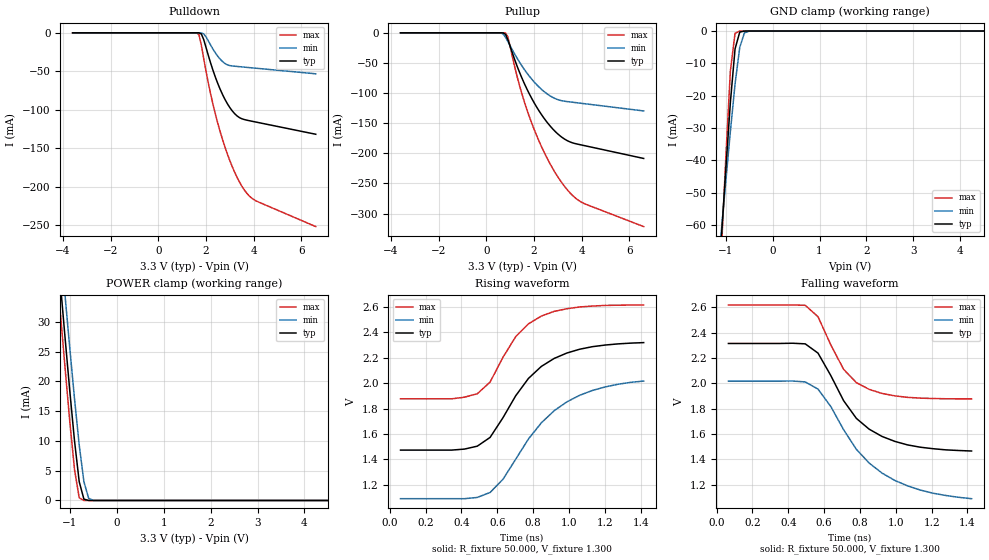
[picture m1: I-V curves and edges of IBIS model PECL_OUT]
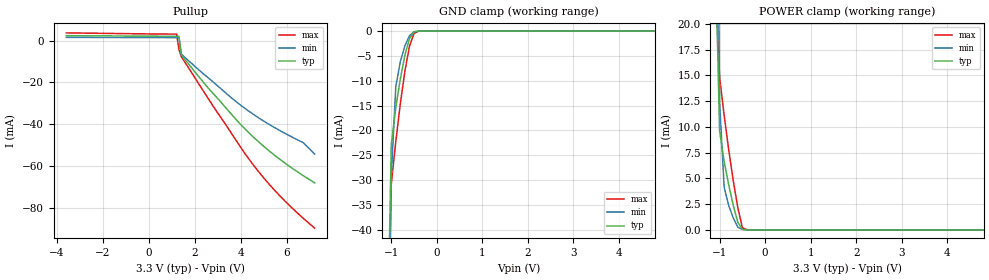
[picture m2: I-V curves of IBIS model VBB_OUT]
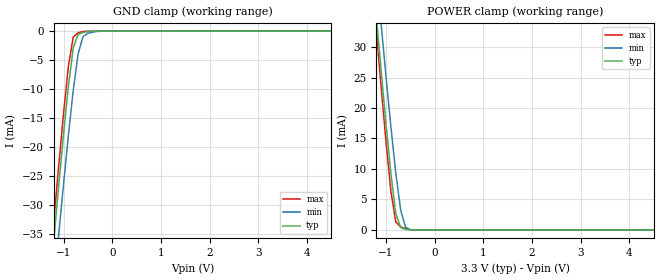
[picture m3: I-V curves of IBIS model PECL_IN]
|   This file is an IBIS representation of the   |
|   Texas Instruments   |
|   CDCP1803   |
|   24-pin MLF Package   |
[IBIS Ver]   3.2
[File name]   cdcp1803.ibs
[File Rev]   1.6
[Date]   1st of March 2005
[Source]   file originated at Texas Instruments
[Notes]   The following information corresponds to the
|   CDCP1803 i/o buffers and input ESD structures.
|Revision log: 0.1, 06/03/2003 file released by TEXAS INSTRUMENTS.
|   1- initial version
|   0.2, 02/06/2004 aligned with final data sheet for CDCP1803
|   0.3, 02/17/2004 corrected Cin/Cout for PECL outputs according
|   to data sheet. Corrected Vinl, Vinh for control input.
|   0.4, 02/18/2004 replaced GND clamp (referenced to VDD) by same
|   plot referenced to GND (0V).
|   0.5, 03/01/2005 added VBB plot.
|   Warnings for VT/IV voltage difference relate to truncated
|   VT plots to allow faster simulation frequency if
|   VT time delay is enabled, which is strongly recommended for
|   correct results of the differential PECL buffers. If this is not
|   required, some simulators require to completely disable use of
|   the VT table for better results. If you note problems with
|   differential cross point, it might point to this situation
|   1.6  06/14/2010 Corrected PECL_OUT warnings for Rising and
|   falling waveforms
[Disclaimer]
(C) Copyright Texas Instruments Incorporated 2004
   All rights reserved
  Texas Instruments Incorporated hereby grants the user of this IBIS
model a non-exclusive, nontransferable license to use this IBIS model
under the following terms.  Before using this IBIS model, the user
should read this license.  If the user does not accept these terms,
the IBIS model should be returned to Texas Instruments within 30 days.
  The user is granted this license only to use the IBIS model and
is not granted rights to sell, load, rent, lease or license the IBIS
model in whole or in part, or in modified form to anyone other than
user.  User may modify the IBIS model to suit its specific applications
but rights to derivative works and such modifications shall belong to
Texas Instruments.
  This IBIS model is provided on an "AS IS" basis and Texas Instruments
makes absolutely no warranty with respect to the information contained
herein.  TEXAS INSTRUMENTS DISCLAIMS AND CUSTOMER WAIVES ALL WARRANTIES,
EXPRESS OR IMPLIED, INCLUDING WARRANTIES OF MERCHANTABILITY OR FITNESS
FOR A PARTICULAR PURPOSE. The entire risk as to quality and performance
is with the Customer. ACCORDINGLY, IN NO EVENT SHALL THE COMPANY BE LIABLE
FOR ANY DAMAGES, WHETHER IN CONTRACT OR TORT,INCLUDING ANY LOST PROFITS
OR OTHER INCIDENTAL, CONSEQUENTIAL, EXEMPLARY, OR PUNITIVE DAMAGES ARISING
OUT OF THE USE OR APPLICATION OF THE IBIS model provided in this package.
Further, Texas Instruments reserves the right to discontinue or make changes
without notice to any product herein to improve reliability, function, or
design. Texas Instruments does not convey any license under patent rights
or any other intellectual property rights, including those of third parties.
Contact Texas Instruments at ATTN: HPA Department,
12500 TI blvd, M/S 8730, Dallas, TX 75243
IBIS Open Forum disclaims all warranties. See DISCLAIM.TXT
in vhdl.org:/pub/IBIS/models for the full disclaimer.
[Copyright]   Copyright 2004, Texas Instruments, All Rights Reserved
[Component]   CDCP1803RTH
[Manufacturer]  Texas Instruments Incorporated
[Package]
|   TYP   MIN   MAX
R_pkg   0.260   0.150   0.310
L_pkg   1.150nH   0.220nH   1.370nH
C_pkg   0.041pF   0.027pF   0.047pF
[Pin]   signal_name   model_name   R_Pin   L_Pin   C_Pin
1   EN   CTRL_IN   0.167ohms   0.683nH   0.028pF
2   VDD   POWER   0.130ohms   0.600nH   0.080pF
3   IN   PECL_IN   0.285ohms   1.249nH   0.044pF
4   INB   PECL_IN   0.270ohms   1.176nH   0.041pF
5   VDD   POWER   0.130ohms   0.600nH   0.080pF
6   VBB   VBB_OUT   0.279ohms   1.221nH   0.044pF
7   VSS   GND   0.050ohms   0.220nH   0.240pF
8   VDD   POWER   0.130ohms   0.600nH   0.080pF
9   Y2   PECL_OUT   0.285ohms   1.250nH   0.044pF
10   Y2B   PECL_OUT   0.270ohms   1.177nH   0.041pF
11   VDD   POWER   0.130ohms   0.600nH   0.080pF
|12   NC   NC   0.302ohms   1.331nH   0.045pF
13   VSS   POWER   0.130ohms   0.600nH   0.080pF
14   VDD   POWER   0.130ohms   0.600nH   0.080pF
15   Y1   PECL_OUT   0.270ohms   1.176nH   0.041pF
16   Y1B   PECL_OUT   0.268ohms   1.166nH   0.041pF
17   VDD   POWER   0.130ohms   0.600nH   0.080pF
18   S0   CTRL_IN   0.302ohms   1.331nH   0.045pF
19   S1   CTRL_IN   0.302ohms   1.331nH   0.045pF
20   VDD   POWER   0.130ohms   0.600nH   0.080pF
21   Y0   PECL_OUT   0.270ohms   1.177nH   0.041pF
22   Y0B   PECL_OUT   0.157ohms   0.641nH   0.027pF
23   VDD   POWER   0.130ohms   0.600nH   0.080pF
24   S2   CTRL_IN   0.167ohms   0.683nH   0.028pF
[Diff_Pin]  inv_pin  vdiff   tdelay_typ  tdelay_min  tdelay_max
3   4   0.5V   0ns   0n   0ns   | IN / INB
9   10   0V   0ns   0ns   0ns   | Y2 / Y2B
15   16   0V   0ns   0ns   0ns   | Y1 / Y1B
21   22   0V   0ns   0ns   0ns   | Y0 / Y0B
| Models and submodels in the file (4): PECL_OUT (3-state_ECL), VBB_OUT (Terminator), PECL_IN (Input), CTRL_IN (Input)
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|   Differential Output Driver MODEL
[Model]   PECL_OUT
Model_type   3-state_ECL
| Signals   Y0, Y0B, Y1, Y1B, Y2, Y2B,
Vmeas = 1.89V   |Vref for timing measurments
Cref = 0pF   |c_load for timing spec
Rref = 50   |R_load for timing spec
Vref = 1.3V   |Timing spec test load voltage
| variable   typ   min   max
C_comp   0.76pF   NA   NA
[Temperature Range]   27   125   -20
[Voltage range]   3.3V   3.0V   3.6V
[Pulldown reference]   3.3V   3.0V   3.6V
[GND Clamp reference]   0V   0V   0V
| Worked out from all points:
|   GND clamp passes 1 mA (typ) near -0.71 V on its own axis
|   POWER clamp passes 1 mA (typ) near -0.73 V on its own axis
|   rising waveform, R_fixture 50.000, V_fixture 1.300: 20-80 % time 275ps typ, 320ps min, 210ps max; typ from 1.47 V to 2.32 V
|   falling waveform, R_fixture 50.000, V_fixture 1.300: 20-80 % time 251ps typ, 314ps min, 183ps max; typ from 2.31 V to 1.47 V
[Pullup]
|   27C:3.3V:nominal   125C:3.0V:weak   -20C:3.6V:strong
|  Voltage   I(typ)   I(min)   I(max)
-3.6V     437pA      8.06nA     324.7pA
500mV     -84.04nA   -11.65uA   -371.3pA
700mV     -101.2uA   -1.872mA   -2.864uA
800mV     -2.246mA   -7.123mA   -226.3uA
900mV     -11.06mA   -14.21mA   -6.425mA
1.4V      -66.31mA   -49.24mA   -88.69mA
1.9V      -108.6mA   -76.68mA   -149.5mA
2.5V      -146mA     -99.87mA   -204.2mA
3.2V      -174.2mA   -112.9mA   -250.6mA
3.6V      -182.4mA   -115.1mA   -269.2mA
4V        -186.2mA   -117mA     -281.2mA
6.6V      -208.5mA   -129.6mA   -321.5mA
[Pulldown]
|   27C:3.3V:nominal   125C:3.0V:weak   -20C:3.6V:strong
|   Voltage   I(typ)   I(min)   I(max)
-3.6V     280.9pA    304.5pA    264.7pA
1.6V      -1.679uA   -521.3nA   -43.83uA
1.7V      -58.05uA   -8.476uA   -2.396mA
1.8V      -1.47mA    -132uA     -16mA
1.9V      -8.843mA   -1.407mA   -33.6mA
2.2V      -40.32mA   -16.53mA   -81.03mA
2.5V      -66.73mA   -30.89mA   -118.8mA
3V        -97.48mA   -42.66mA   -166.6mA
3.5V      -111.8mA   -44.34mA   -199.5mA
3.8V      -114.3mA   -45.21mA   -211.9mA
4.1V      -116.2mA   -46.08mA   -218.7mA
6.6V      -132mA     -53.32mA   -252.1mA
[GND Clamp]
|   27C:3.3V:nominal   125C:3.0V:weak   -20C:3.6V:strong
|   Voltage   I(typ)   I(min)   I(max)
-3.6V     -846.1mA   -726mA     -1.01A
-1.1V     -65.74mA   -63.12mA   -70.56mA
-1V       -43.58mA   -46.98mA   -40.08mA
-900mV    -22.15mA   -31.16mA   -12.38mA
-800mV    -5.529mA   -16.41mA   -692.9uA
-700mV    -333.5uA   -5.056mA   -8.688uA
-600mV    -9.161uA   -575uA     -94.39nA
-500mV    -237.2nA   -35.55uA   -1.21nA
6.6V      452.4pA    471.7pA    424.6pA
[POWER Clamp]
|   27C:3.3V:nominal   125C:3.0V:weak   -20C:3.6V:strong
|  Voltage   I(typ)   I(min)   I(max)
-3.6V     263.5mA    264.3mA    263.5mA
-1.3V     45.57mA    52.26mA    40.83mA
-1.2V     36.3mA     43.2mA     31.38mA
-1.1V     27.17mA    34.25mA    22.11mA
-1V       18.31mA    25.49mA    13.19mA
-900mV    9.992mA    17.07mA    5.178mA
-800mV    3.144mA    9.308mA    454.2uA
-700mV    228.8uA    3.147mA    5.697uA
-600mV    6.116uA    387.4uA    58.55nA
-500mV    150.9nA    23.42uA    752.7pA
6.6V      0A         0A         0A
[ramp]
| variable   typ   min   max
dV/dt_r   0.5117/2.7842E-10   0.5571/3.3895E-10   0.4456/2.0819E-10
dV/dt_f   0.5117/2.5529E-10   0.5571/3.4568E-10   0.4456/1.8152E-10
[Rising Waveform]
R_fixture = 50.000
V_fixture = 1.300
V_fixture_min = 1.000
V_fixture_max = 1.600
|  time   V(typ)   V(min)   V(max)
59.71ps   1.473V     1.09V      1.877V
416.9ps   1.481V     1.09V      1.89V
488.3ps   1.504V     1.1V       1.917V
559.7ps   1.573V     1.139V     2.009V
631.1ps   1.727V     1.242V     2.203V
702.6ps   1.901V     1.401V     2.367V
845.4ps   2.132V     1.687V     2.529V
916.9ps   2.195V     1.783V     2.566V
1.06ns    2.268V     1.905V     2.601V
1.417ns   2.32V      2.017V     2.617V
[Falling Waveform]
R_fixture = 50.000
V_fixture = 1.300
V_fixture_min = 1.000
V_fixture_max = 1.600
|  time   V(typ)   V(min)   V(max)
65.71ps   2.314V     2.017V     2.617V
494.3ps   2.311V     2.011V     2.615V
565.7ps   2.238V     1.954V     2.525V
637.1ps   2.061V     1.817V     2.303V
708.6ps   1.863V     1.634V     2.11V
780ps     1.723V     1.479V     2.005V
851.4ps   1.638V     1.371V     1.952V
994.3ps   1.542V     1.234V     1.901V
1.209ns   1.484V     1.133V     1.88V
1.423ns   1.466V     1.09V      1.877V
[Model]   VBB_OUT
Model_type   Terminator
| Signals   VBB
| variable   typ   min   max
C_comp   3pF   NA   NA
[Temperature Range]   27   125   -20
[Voltage range]   3.3V   3.0V   3.6V
[Pulldown reference]   3.3V   3.0V   3.6V
[GND Clamp reference]   0V   0V   0V
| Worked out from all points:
|   slope of the pullup table from 0 to 0.3 V, typ, clamps not added: 17.1 kohm
|   GND clamp passes 1 mA (typ) near -0.56 V on its own axis
|   POWER clamp passes 1 mA (typ) near -0.62 V on its own axis
[Pullup]
|   27C:3.3V:nominal   125C:3.0V:weak   -20C:3.6V:strong
|  Voltage   I(typ)   I(min)   I(max)
-3.6V     2.446mA    1.631mA    3.77mA
1.2V      2.141mA    1.477mA    3.181mA
1.3V      2.136mA    1.473mA    -4.215mA
1.4V      -6.876mA   -6.326mA   -7.569mA
2.6V      -23mA      -18.01mA   -28.17mA
3.6V      -35.46mA   -27.52mA   -44.68mA
4.2V      -42.58mA   -32.66mA   -54.52mA
4.9V      -49.79mA   -37.9mA    -64.6mA
5.5V      -55.23mA   -41.88mA   -72.15mA
6.1V      -60.14mA   -45.49mA   -78.91mA
6.7V      -64.61mA   -48.82mA   -85.04mA
7.2V      -68.11mA   -54.32mA   -89.82mA
[Pulldown]
|   27C:3.3V:nominal   125C:3.0V:weak   -20C:3.6V:strong
|   Voltage   I(typ)   I(min)   I(max)
-3.6V     0A         0A         0A
7.2V      0A         0A         0A
[GND Clamp]
|   27C:3.3V:nominal   125C:3.0V:weak   -20C:3.6V:strong
|   Voltage   I(typ)   I(min)   I(max)
-3.6V     -2.087A    -1.713A    -2.549A
-1.2V     -121.5mA   -139.6mA   -120.3mA
-1V       -22.85mA   -29.28mA   -30.78mA
-900mV    -15.35mA   -11.09mA   -22.19mA
-800mV    -9.579mA   -6.1mA     -14.55mA
-700mV    -4.815mA   -2.942mA   -8.017mA
-600mV    -1.516mA   -928.7uA   -3.052mA
-500mV    -179.1uA   -134uA     -460uA
-400mV    0A         0A         0A
7.2V      0A         0A         0A
[POWER Clamp]
|   27C:3.3V:nominal   125C:3.0V:weak   -20C:3.6V:strong
|  Voltage   I(typ)   I(min)   I(max)
-3.7V     3.647A     3.064A     4.328A
-1.1V     28.23mA    63.25mA    24.27mA
-1V       9.616mA    12.37mA    14.85mA
-900mV    6.652mA    4.149mA    11.13mA
-800mV    4.373mA    2.372mA    7.786mA
-700mV    2.384mA    1.169mA    4.777mA
-600mV    747.3uA    271.7uA    2.165mA
-500mV    71.53uA    50.13uA    220.1uA
-400mV    15.38uA    11.13uA    35.72uA
-100mV    196.4nA    62.93nA    440.9nA
7.2V      0A         0A         0A
|   Differential Input Receiver Model
[Model]   PECL_IN
Model_type   Input
Polarity   Non-Inverting
Enable   Active-High
Vinl = 1.6575V   | PECL levels refer to VDD. 3.3-(1.81+1.475)/2
Vinh = 2.2775V   |   3.3-(1.165+.088)/2
|   typ   min   max
C_comp   0.76pF   NA   NA
[Temperature range]   27   125   -20
[Voltage range]   3.3   3.0   3.6
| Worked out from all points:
|   GND clamp passes 1 mA (typ) near -0.72 V on its own axis
|   POWER clamp passes 1 mA (typ) near -0.73 V on its own axis
| Notes: (1) Vtable = Vcc - Voutput
|   (2) Pullup data includes the effects of the clamping circuitry
[POWER Clamp]
|   27C:3.3V:nominal   125C:3.0V:weak   -20C:3.6V:strong
|  Voltage   I(typ)   I(min)   I(max)
-3.6V     265.8mA    263.4mA    273.1mA
-1.2V     35.02mA    42.56mA    32.64mA
-1.1V     26mA       33.7mA     23.35mA
-1V       17.28mA    25.09mA    14.39mA
-900mV    9.15mA     16.88mA    6.291mA
-800mV    2.691mA    9.338mA    1.306mA
-700mV    397uA      3.282mA    517.8uA
-600mV    106.3uA    454.8uA    227uA
-500mV    15.87uA    36.77uA    48.73uA
6.6V      0A         0A         0A
[GND Clamp]
|   27C:3.3V:nominal   125C:3.0V:weak   -20C:3.6V:strong
|  Voltage   I(typ)   I(min)   I(max)
-3.6V     -268.1mA   -268.4mA   -271.2mA
-1.3V     -45.38mA   -53.26mA   -42.38mA
-1.2V     -35.99mA   -44.19mA   -32.76mA
-1.1V     -26.76mA   -35.23mA   -23.31mA
-1V       -17.81mA   -26.44mA   -14.21mA
-900mV    -9.461mA   -17.98mA   -5.998mA
-800mV    -2.874mA   -10.17mA   -1.017mA
-700mV    -575.1uA   -3.894mA   -292.2uA
-600mV    -252.8uA   -947.5uA   -69.37uA
-500mV    -74.55uA   -385.7uA   -9.282uA
-300mV    -10.26uA   -59.25uA   -7.753uA
6.6V      0A         0A         0A
